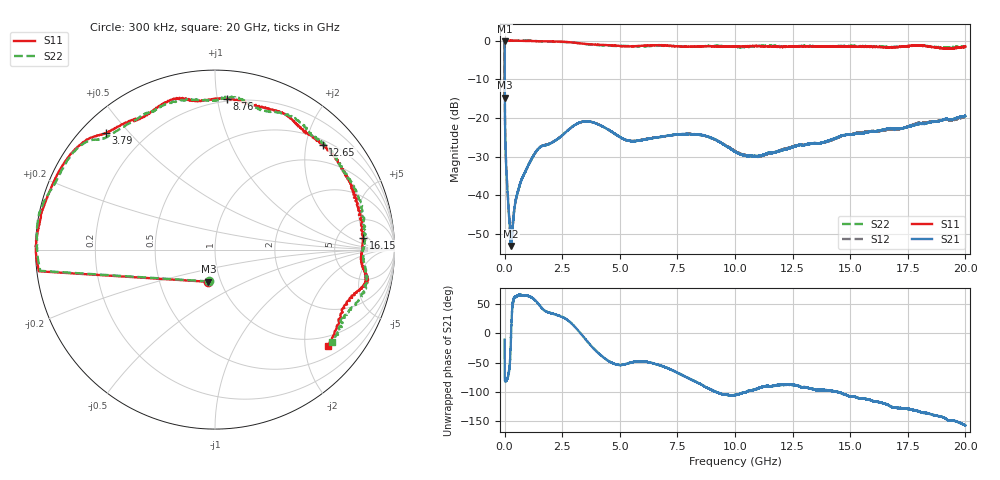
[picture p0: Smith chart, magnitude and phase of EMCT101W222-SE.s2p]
!EMCT101W222
!Johanson Technology Inc.
!www.johansontechnology.com
!Test Board Conditions:
!Substrate Type  RO4350B
!Substrate Thickness  10 mil
!Substrate Dk  3.66
!TL Type: GCPW
!TL Trace Width  22 mil
!TL Gap  14 mil
!PART MODE SINGLE ENDED (AKA BYPASS)
!DUT TOPOLOGY	SERIES-SHUNT
# MHz S  dB  R 50
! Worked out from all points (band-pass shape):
!   20001 points, 300 kHz to 20 GHz, reference 50 ohm
!   highest |S21| = -0.18 dB at 300 kHz (marker M1); lowest = -53.1 dB at 282.3 MHz (marker M2)
!   |S21| within 3 dB of the highest: start of sweep to 1.647 MHz
!   lowest |S11| = -14.7 dB at 300 kHz (marker M3), VSWR 1.45, Z = 43.7 - j16.2 ohm
!   |S11| at or under -10 dB: start of sweep to 744.8 kHz
!   |S22| runs from -14.9 to 0.0 dB; largest |S21 - S12| = 0.0058
!   S11 on the Smith chart (normalised r, x): 300 kHz: 0.87, -0.32; 3.79 GHz: 0.07, +0.43; 8.76 GHz: 0.18, +1.06; 12.65 GHz: 0.59, +2.33; 16.15 GHz: 9.07, +3.81; 20 GHz: 0.71, -2.52
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0.3  -14.74 -101.5  -0.18 -10.8  -0.18 -10.8  -14.85 -101.4
101.298  -0.01 179.9  -36.38 -79.8  -36.38 -79.8  -0.09 -180.0
123.298  -0.02 179.5  -38.61 -77.6  -38.55 -77.5  -0.07 179.7
208.297  -0.02 178.5  -46.65 -58.8  -46.44 -59.6  -0.07 178.3
282.296  -0.02 177.6  -53.10 -1.8  -52.11 -2.4  -0.05 177.2
644.29  -0.07 173.6  -37.58 66.3  -37.65 66.2  -0.01 172.6
1308.28  -0.16 164.9  -29.23 57.5  -29.24 58.0  -0.12 163.6
3334.25  -0.76 136.2  -21.07 -1.5  -21.08 -1.5  -0.77 138.1
3790.243  -1.01 133.2  -21.09 -22.7  -21.09 -22.8  -1.07 136.0
5338.22  -1.51 118.7  -25.85 -51.9  -25.87 -51.3  -1.40 116.5
6667.2  -1.22 105.4  -25.03 -53.9  -25.00 -54.4  -1.37 109.4
8760.169  -1.49 85.5  -24.72 -92.8  -24.76 -93.1  -1.47 87.0
10000.15  -1.57 71.0  -28.75 -105.6  -28.60 -105.8  -1.70 74.0
11054.13  -1.44 61.4  -29.91 -93.1  -29.97 -94.2  -1.40 63.3
12654.11  -1.53 44.2  -27.21 -89.1  -27.21 -89.5  -1.44 45.6
13334.1  -1.52 34.9  -26.71 -95.1  -26.62 -95.3  -1.47 37.5
15024.08  -1.59 21.5  -24.32 -108.3  -24.27 -106.7  -1.41 19.1
16154.06  -1.63 4.5  -23.41 -117.2  -23.47 -119.1  -1.53 4.7
16667.05  -1.75 -1.9  -22.75 -123.6  -22.96 -123.1  -1.66 0.4
18031.03  -1.38 -12.9  -21.53 -134.5  -21.32 -134.9  -1.36 -15.3
19172.01  -2.05 -24.2  -20.24 -147.0  -20.39 -148.8  -1.84 -28.9
20000  -1.60 -40.7  -19.51 -158.1  -19.72 -155.8  -1.57 -38.4
